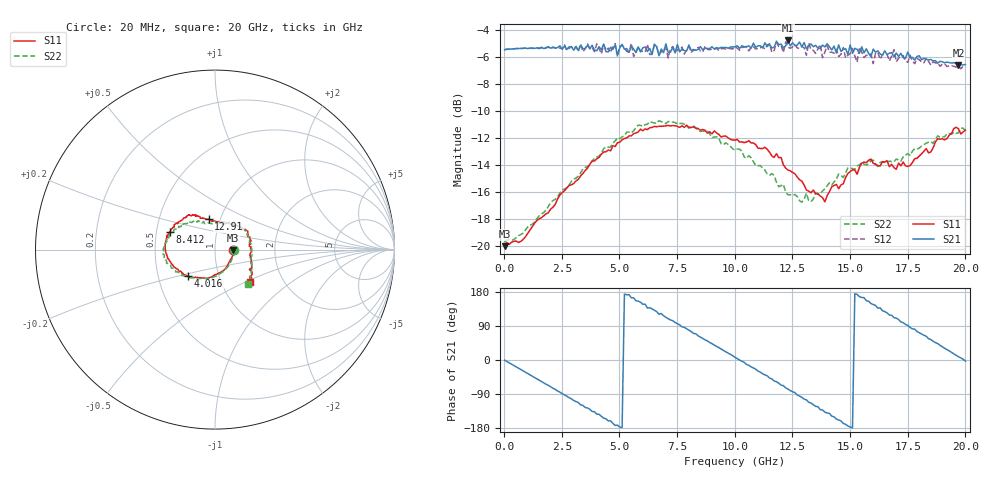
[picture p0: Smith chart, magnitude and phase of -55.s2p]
!Agilent Technologies,N5230A,US43500223,A.07.50.48
!Agilent N5230A: A.07.50.48
!Date: Saturday, September 19, 2015 14:42:01
!Correction: S11(Full 2 Port(1,2))
!S21(Full 2 Port(1,2))
!S12(Full 2 Port(1,2))
!S22(Full 2 Port(1,2))
!S2P File: Measurements: S11, S21, S12, S22:
# Hz S  dB  R 50
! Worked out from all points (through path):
!   201 points, 20 MHz to 20 GHz, reference 50 ohm
!   highest |S21| = -4.79 dB at 12.31 GHz (marker M1); lowest = -6.6 dB at 19.7 GHz (marker M2)
!   group delay of S21, straight-line fit = 100 ps
!   lowest |S11| = -20.0 dB at 20 MHz (marker M3), VSWR 1.22, Z = 61.1 - j0.365 ohm
!   |S11| at or under -10 dB: start of sweep to end of sweep
!   |S22| runs from -19.7 to -10.7 dB; largest |S21 - S12| = 0.079
!   S11 on the Smith chart (normalised r, x): 20 MHz: 1.22, -0.01; 4.016 GHz: 0.71, -0.22; 8.412 GHz: 0.59, +0.13; 12.91 GHz: 0.88, +0.31; 20 GHz: 1.37, -0.54
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2e7  -20.03 -1.7  -5.47 -0.6  -5.47 -0.7  -19.71 -1.3
9.191e8  -19.34 -45.6  -5.35 -31.8  -5.35 -32.1  -18.85 -44.4
1.9181e9  -17.55 -81.2  -5.28 -67.0  -5.24 -67.4  -17.06 -80.4
3.4166e9  -14.64 -123.4  -5.39 -120.0  -5.61 -122.1  -14.31 -120.1
4.016e9  -13.56 -134.9  -5.55 -142.9  -5.03 -144.0  -13.43 -133.8
5.1149e9  -12.14 -157.1  -5.07 -178.1  -5.16 -179.7  -11.94 -153.9
6.1139e9  -11.33 -172.9  -5.27 147.3  -5.65 147.3  -11.02 -168.2
6.7133e9  -11.14 179.3  -5.91 120.7  -5.87 120.0  -10.73 -174.5
7.5125e9  -11.15 169.9  -5.08 95.7  -5.47 96.0  -10.98 176.6
8.4116e9  -11.31 158.6  -5.44 63.8  -5.29 61.4  -11.43 166.7
1.001e10  -12.17 136.6  -5.25 7.0  -5.26 5.2  -12.91 141.5
1.13087e10  -12.70 122.6  -4.96 -39.2  -5.43 -39.6  -14.38 125.4
1.23077e10  -14.38 114.1  -4.79 -76.7  -5.29 -79.8  -16.22 110.6
1.29071e10  -15.20 102.0  -5.25 -98.5  -5.23 -102.0  -16.77 95.4
1.34066e10  -15.87 92.4  -5.25 -118.0  -5.52 -122.5  -16.53 82.7
1.5005e10  -14.50 43.4  -5.12 -177.0  -5.76 -174.2  -14.23 40.1
1.54046e10  -14.19 35.6  -5.74 167.4  -5.31 169.5  -14.02 30.1
1.67033e10  -14.13 11.8  -5.72 118.9  -6.31 119.1  -13.71 -1.4
1.79021e10  -13.52 -17.3  -5.97 75.3  -6.11 75.8  -12.83 -26.8
1.88012e10  -12.07 -33.9  -6.46 43.3  -6.46 38.9  -11.85 -39.1
1.97003e10  -11.33 -43.8  -6.60 8.7  -6.71 6.2  -11.62 -45.0
2e10  -11.42 -42.6  -6.57 -3.0  -6.73 -5.7  -11.48 -45.9
